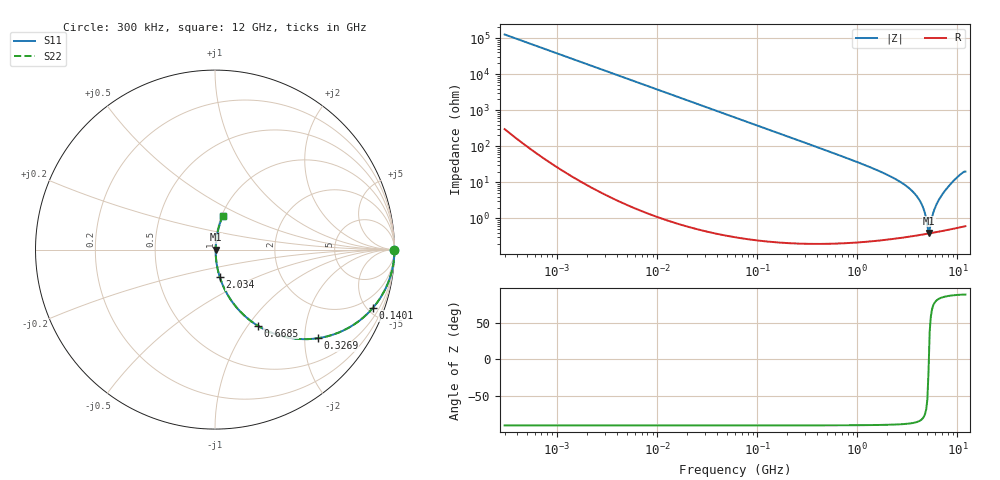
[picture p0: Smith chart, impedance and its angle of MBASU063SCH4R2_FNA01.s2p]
! MBASU063SCH4R2_FNA01  S-PARAMETER MODEL  ( General Type )
! Model Generated by TAIYO YUDEN Corporation (http://www.ty-top.com)
! Version 1.0
! TAIYO YUDEN Control No. 130801
! Copyright(c) 2013 TAIYO YUDEN CO.,LTD. All Rights Reserved.
! Product Description (link to TY-COMPAS)
! https://ds.yuden.co.jp/TYCOMPAS/or/detail?pn=MBASU063SCH4R2CFNA01&u=M
! Products Name : Multilayer Ceramic Capacitors
! Characteristics :
!  Capacitance : 4.2 pF , Rated Voltage : 50V , TCC : CH / C0H
!  Case Size : 0.6 x 0.3 / 0.024 x 0.012 [mm/inch] , Thickness : 0.3 / 0.012 [mm/inch]
!  (Conditions: Temperature = 25 degC , DC Bias Current/Voltage = 0A / 0V)
! External Node Assignments :
!  1  o---| |---o  2
! GND o---------o GND
! Frequency Range : 0.3MHz  -  12000MHz  [ 401 STEP ]
# MHz S RI R 50
! Freq[MHz].  S11 Real  S11 Imag  S21 Real  S21 Imag  S12 Real  S12 Imag  S22 Real  S22 Imag
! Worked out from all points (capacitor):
!   401 points, 300 kHz to 12 GHz, reference 50 ohm
!   read as one part in series: C = 4.2 pF near 316.3 kHz
!   lowest |Z| = 398 mohm at 5.141 GHz (marker M1)
!   series resonance near 5.178 GHz, so ESL is about 220 pH
!   S11 on the Smith chart (normalised r, x): 300 kHz: open; 140.1 MHz: 1.00, -5.41; 326.9 MHz: 1.00, -2.31; 668.5 MHz: 1.00, -1.11; 2.034 GHz: 1.01, -0.32; 12 GHz: 1.01, +0.40
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0.3  1 -0.000792  2.51e-06 0.000792  2.51e-06 0.000792  1 -0.000792
1.769972  1 -0.00467  2.4e-05 0.00467  2.4e-05 0.00467  1 -0.00467
10.44266  0.9992 -0.0275  0.000767 0.0275  0.000767 0.0275  0.9992 -0.0275
60  0.9755 -0.1544  0.0245 0.1544  0.0245 0.1544  0.9755 -0.1544
140.0606  0.8795 -0.3252  0.1205 0.3252  0.1205 0.3252  0.8795 -0.3252
326.9496  0.5712 -0.494  0.4288 0.494  0.4288 0.494  0.5712 -0.494
353.9943  0.5317 -0.4981  0.4683 0.4981  0.4683 0.4981  0.5317 -0.4981
668.5285  0.2379 -0.424  0.7621 0.424  0.7621 0.424  0.2379 -0.424
1105.905  0.0983 -0.2943  0.9017 0.2943  0.9017 0.2943  0.0983 -0.2943
2033.931  0.0267 -0.1531  0.9733 0.1531  0.9733 0.1531  0.0267 -0.1531
2088.533  0.0251 -0.1479  0.9749 0.1479  0.9749 0.1479  0.0251 -0.1479
3026.31  0.00973 -0.0816  0.9903 0.0816  0.9903 0.0816  0.00973 -0.0816
3841.137  0.00529 -0.0443  0.9947 0.0443  0.9947 0.0443  0.00529 -0.0443
4502.883  0.004 -0.0207  0.996 0.0207  0.996 0.0207  0.004 -0.0207
5006.236  0.00378 -0.00525  0.9962 0.00525  0.9962 0.00525  0.00378 -0.00525
5140.631  0.00381 -0.0011  0.9962 0.0011  0.9962 0.0011  0.00381 -0.0011
5420.343  0.00394 0.0063  0.9961 -0.0063  0.9961 -0.0063  0.00394 0.0063
5868.704  0.00435 0.0169  0.9956 -0.0169  0.9956 -0.0169  0.00435 0.0169
6188.031  0.00478 0.0244  0.9952 -0.0244  0.9952 -0.0244  0.00478 0.0244
7064.448  0.0066 0.0459  0.9934 -0.0459  0.9934 -0.0459  0.0066 0.0459
9454.42  0.0196 0.1184  0.9804 -0.1184  0.9804 -0.1184  0.0196 0.1184
12000  0.0436 0.1894  0.9564 -0.1894  0.9564 -0.1894  0.0436 0.1894
